// TwinCAT 3 PLC project Untitled1
// ProgramVersion: 3.1.4026.17
// libraries:
//   Tc2_MC2, * (Beckhoff Automation GmbH)
//   Tc2_Standard, * (Beckhoff Automation GmbH)
//   Tc2_System, * (Beckhoff Automation GmbH)
// project tree:
//   DUTs/ ST_axis_Vel.TcDUT
//   / FB_NcAxis.TcPOU, PlcTask.TcTTO
//   POUs/ MAIN.TcPOU
// real-time tasks:
//   TASK PlcTask: cycle T#10ms, priority 20, ADS port 350
// motion (NC):
//   TASK NC-Task 1 SAF: cycle T#2ms, priority 4, ADS port 501
//   TASK NC-Task 1 SVB: cycle T#10ms, priority 8, ADS port 511
//   AXIS NCAxis (id 1)
//     OtherSettings: AllowMotionCmdToSlave=true
//     encoder EncType=1
//     drive DrvType=5
//       Analog: TorqueSetpointScale=10, ScaleFactorActTorque=0.1
//       TimeComp: TaskDelayCycles=1
//     controller CtrType=1
//       CtrPara: PriorControlFactor=1
//         Observer: BandWidth=20
// variable links:
//   Untitled1/Untitled1 Instance <-> NC-Task 1 SAF/Axes/NCAxis
//     PlcTask Inputs/MAIN.Axis.NcToPlc <-> Outputs/ToPlc
//     PlcTask Outputs/MAIN.Axis.PlcToNc <-> Inputs/FromPlc

CONFIGURATION Untitled1
    RESOURCE PLC ON TwinCAT3
        TASK PlcTask(INTERVAL := T#10ms, PRIORITY := 20);
        PROGRAM MAIN WITH PlcTask : MAIN;
    END_RESOURCE
END_CONFIGURATION

// ---- DUTs/ST_axis_Vel.TcDUT
TYPE ST_axis_Vel :
STRUCT
	  Axis_Vel:REAL;  //绝对移动速度
	  Axis_Acc:REAL;  //移动加速度
	  Axis_Dec:REAL;  //移动减速度
	  Axis_Jerk:REAL;//移动加加速度
END_STRUCT
END_TYPE

// ---- POUs/MAIN.TcPOU
PROGRAM MAIN
VAR
	Axis: FB_NcAxis;
END_VAR

Axis.TestMode();

END_PROGRAM

// ---- FB_NcAxis.TcPOU
// 轴对象
FUNCTION_BLOCK FB_NcAxis EXTENDS Tc2_MC2.AXIS_REF 
VAR
	{attribute ‘hide’}
	mcReadStatus	         :Tc2_MC2.MC_ReadStatus;	
	{attribute ‘hide’}
	mcReadActPos	         :Tc2_MC2.MC_ReadActualPosition;
	{attribute ‘hide’}
	mcReadActVel             :Tc2_MC2.MC_ReadActualVelocity;
	{attribute ‘hide’}
	mcPower                  :Tc2_MC2.MC_Power;
	{attribute ‘hide’}
	mcMoveRel		         :Tc2_MC2.MC_MoveRelative;
	{attribute ‘hide’}
	mcMoveAbs		         :Tc2_MC2.MC_MoveAbsolute;
	{attribute ‘hide’}
	mcMoveVelocity           :Tc2_MC2.MC_MoveVelocity;
	{attribute ‘hide’}
	mcMoveModulo			 :Tc2_MC2.MC_MoveModulo;
	{attribute ‘hide’}
	mcReset                  :Tc2_MC2.MC_Reset;
	{attribute ‘hide’}
	mcJogContinous           :Tc2_MC2.MC_Jog;
	{attribute ‘hide’}
	mcJogRelative            :Tc2_MC2.MC_Jog;
	{attribute ‘hide’}
	mcStop                   :Tc2_MC2.MC_Stop;
	{attribute ‘hide’}
	mcHalt                   :Tc2_MC2.MC_Halt;
	{attribute ‘hide’}
	mcsetOverride            :Tc2_MC2.MC_SetOverride;

	mchome					 :Tc2_Mc2.MC_Home;
	
	_NCTOPLC				 : NCTOPLC_AXIS_REF;

	
END_VAR

PROPERTY AxesStatus : REFERENCE TO Tc2_Mc2.ST_AxisStatus
GET
AxesStatus	REF= Status;
END_GET
END_PROPERTY

// 刷新状态
METHOD PUBLIC CyclicCheck
VAR_INPUT
END_VAR
ReadStatus();
_NCTOPLC	:= NCTOPLC;
END_METHOD

// 暂停
METHOD Halt : BOOL
VAR_INPUT
	Execute              :BOOL;
END_VAR
mcHalt(
	Axis:=THIS^ , 
	Execute:=Execute , 
	Deceleration:=800000 , 
	Jerk:=80000 , 
	BufferMode:= , 
	Options:= , 
	Done=> , 
	Busy=> , 
	Active=> , 
	CommandAborted=> , 
	Error=>Status.Error , 
	ErrorID=>Status.ErrorId );
	
IF mcHalt.Done AND NOT Status.Error THEN
	Halt := TRUE;
ELSE
	Halt := FALSE;
END_IF
END_METHOD

// 绝对定位
METHOD MoveAbs : BOOL
VAR_INPUT
	Execute             :BOOL;
	TargetPos:REAL;
	TargetVel         :ST_axis_Vel;
END_VAR
mcMoveAbs(
	Axis:= THIS^, 
	Execute:= Execute, 
	Position:= TargetPos, 
	Velocity:= TargetVel.Axis_Vel, 
	Acceleration:= TargetVel.Axis_Acc, 
	Deceleration:= TargetVel.Axis_Dec, 
	Jerk:= TargetVel.Axis_Jerk, 
	BufferMode:= , 
	Options:= , 
	Done=> , 
	Busy=> , 
	Active=> , 
	CommandAborted=> , 
	Error=>Status.Error , 
	ErrorID=>Status.ErrorId );
	
IF mcMoveAbs.Done AND NOT Status.Error THEN
	MoveAbs := TRUE;
ELSE
	MoveAbs := FALSE;
END_IF
END_METHOD

// 点动
METHOD MoveJog : BOOL
VAR_INPUT
	JogForward                 :BOOL;
	JogBackwards               :BOOL;
	TargetVel       :LREAL;
END_VAR
mcJogContinous(
	JogForward:= 	JogForward,
	JogBackwards:= 	JogBackwards,
	Mode:= 			MC_JOGMODE_CONTINOUS,
	Velocity:= 		TargetVel,
	Axis:= 			THIS^,
	Error=>Status.Error , 
	ErrorID=>Status.ErrorId );
	
MoveJog:=mcJogContinous.Busy;
END_METHOD

// 速度运动
METHOD MoveVelocity : BOOL
VAR_INPUT
	Execute:BOOL;
	TargetVel       : ST_axis_Vel;
	Direction		: MC_Direction;
END_VAR
mcMoveVelocity(
	Axis:=THIS^ , 
	Execute:= Execute, 
	Velocity:= TargetVel.Axis_Vel, 
	Acceleration:= TargetVel.Axis_Acc, 
	Deceleration:= TargetVel.Axis_Dec, 
	Jerk:= TargetVel.Axis_Jerk, 
	Direction:= Direction, 
	BufferMode:= , 
	Options:= , 
	InVelocity=> , 
	Busy=> , 
	Active=> , 
	CommandAborted=> , 
	Error=>Status.Error , 
	ErrorID=> Status.ErrorId);
END_METHOD

PROPERTY NC_TO_PLC : REFERENCE TO Tc2_Mc2.NCTOPLC_AXIS_REF
GET
NC_TO_PLC	REF= _NcToPlc;
END_GET
END_PROPERTY

// 使能
METHOD Power : BOOL
VAR_INPUT
	Enable         :BOOL;
END_VAR
mcPower(
	Axis:= THIS^, 
	Enable:= Enable, 
	Enable_Positive:=TRUE, //NOT AxisSingle.Positive, 
	Enable_Negative:=TRUE, //NOT AxisSingle.Negtive, 
	Error=>Status.Error , 
	ErrorID=>Status.ErrorId );
END_METHOD

PROPERTY rAxis : REFERENCE TO Tc2_Mc2.AXIS_REF
GET
rAxis	REF= THIS^;
END_GET
END_PROPERTY

// 复位
METHOD Reset : BOOL
VAR_INPUT
	Execute              :BOOL;
END_VAR
mcReset(
	Axis:= THIS^, 
	Execute:=Execute , 
	Error=>Status.Error , 
	ErrorID=>Status.ErrorId );
	
IF NOT Status.Error	AND mcReset.Done THEN
	Reset	:= TRUE;
END_IF
END_METHOD

// 停止
METHOD Stop : BOOL
VAR_INPUT
	Execute              :BOOL;
END_VAR
mcStop(
	Axis:= THIS^, 
	Execute:=Execute , 
	Error=>Status.Error , 
	ErrorID=>Status.ErrorId );
	
	
IF NOT Status.Error	AND mcStop.Done THEN
	Stop	:= TRUE;
END_IF
END_METHOD

METHOD TestMode
VAR_INPUT
END_VAR
VAR
	
END_VAR
THIS^.CyclicCheck();

mcPower(
	Axis:= THIS^,
	Enable_Positive:=TRUE,
	Enable_Negative:=TRUE );
	
mcMoveAbs(Axis:= THIS^ );

mcReset(Axis:= THIS^);

mcStop(Axis:= THIS^);
END_METHOD

END_FUNCTION_BLOCK
